|   IBIS model for TI AM261
[IBIS Ver]   5.1
[Disclaimer]   Please be aware that in the absence of a written agreement
|   Texas Instruments(TI) assumes no liability for:
|   (1) The accuracy of the IBIS models provided to your company,
|   however, the IBIS model is compliant to industry standard
|   IQ Level 2a.  Refer to IBIS Quality Section below for
|   for full details.
|   (2) The proper functioning of these Models in your design
|   or for any resulting applications
|   (3) Infringement of patents, copyrights or intellectual
|   property rights resulting from your use of these
|   models.
|   TI provides IBIS Models as a service to our customers and
|   therefore reserves the right to limit distribution of the
|   Models.  The information is subject to change without notice.
[File Name]  zfg.ibs
[File Rev]   0.1
|   -Initial version
|   -Updated Package model
[Date]   10 October 2024
[Source]   Texas Instruments Incorporated
[Copyright]   Property of Texas Instruments Incorporated.
|   Unauthorized reproduction and/or distribution is strictly.
|   prohibited.
|   This product is protected under copyright law and trade
|   secret law as an unpublished work.
|   Created 2012,(C) Copyright 1999-2012,
|   Texas Instruments Incorporated., All Rights Reserved.
|   These commodities are under the U.S. Government
|   distribution license control. As such,they are not to be
|   re-exported without the prior approval of the U.S.
|   Department of Commerce.
[Notes]
   ADC pins are marked as NC
   USB pins are marked as NC
   Clock pins are marked as NC
   nReset pin marked as NC
|   Revision History
|   GERNERAL COMMENT: All IBIS Quality Notes below reflect latest release
|   and version of IBIS File
|   File passes ibischk6.0 with 0 errors and 35 warnings
|   Component AM261
[Component] AM261
[Manufacturer] TEXAS INSTRUMENTS
[Package Model] AM261_ZFG
[Package]
|   typ   min   max
R_pkg   0.18633   0.087237   0.33822
L_pkg   3.165e-9   1.403e-9   5.371e-9
C_pkg   4.685e-13   3.303e-13   9.903e-13
[Pin]   Signal_name   model_name
F7   VDD   POWER
F9   VDD   POWER
F12   VDD   POWER
F14   VDD   POWER
G6   VDD   POWER
G15   VDD   POWER
J6   VDD   POWER
J15   VDD   POWER
M6   VDD   POWER
M15   VDD   POWER
P6   VDD   POWER
P15   VDD   POWER
R7   VDD   POWER
U10   VDDA18_LDO   POWER
U11   VDDA18_LDO   POWER
U8   VDDA18_OSC_PLL   POWER
T5   VDDA18_USB   POWER
T9   VDDA33   POWER
T12   VDDA33   POWER
P5   VDDA33_USB   POWER
D13   VDDAR2   POWER
H4   VDDAR3   POWER
E9   VDDS18   POWER
E14   VDDS18   POWER
F4   VDDS18   POWER
G16   VDDS18   POWER
L17   VDDS18   POWER
N4   VDDS18   POWER
T16   VDDS18   POWER
U6   VDDS18_LDO   POWER
E7   VDDSHV_A   POWER
E12   VDDSHV_A   POWER
E16   VDDSHV_A   POWER
G5   VDDSHV_A   POWER
J16   VDDSHV_A   POWER
M16   VDDSHV_A   POWER
M5   VDDSHV_B   POWER
T14   VDDSHV_C   POWER
J5   VDDSHV_D   POWER
P16   VDDSHV_E   POWER
T7   VDDSHV_F   POWER
V7   VDD_TEMP   NC
K17   VNWA   POWER
P3   VPP   POWER
W13   ADC0_AIN0   NC
U13   ADC0_AIN1   NC
W14   ADC0_AIN2   NC
V14   ADC0_AIN3   NC
Y14   ADC0_AIN4   NC
W15   ADC0_AIN5   NC
Y15   ADC0_AIN6   NC
W12   ADC1_AIN0   NC
V12   ADC1_AIN1   NC
Y11   ADC1_AIN2   NC
W11   ADC1_AIN3   NC
Y10   ADC1_AIN4   NC
W10   ADC1_AIN5   NC
W9   ADC1_AIN6   NC
W8   ADC2_AIN0   NC
Y7   ADC2_AIN1   NC
Y6   ADC2_AIN2   NC
W7   ADC2_AIN3   NC
W6   ADC2_AIN4   NC
V9   ADC2_AIN5   NC
Y5   ADC2_AIN6   NC
V16   ADC_CAL0   NC
Y12   ADC_VREFHI_G0   NC
Y8   ADC_VREFHI_G1   NC
Y13   ADC_VREFLO_G0   NC
Y9   ADC_VREFLO_G1   NC
W5   ATESTV1   NC
W4   DAC_OUT   NC
U15   DAC_VREF0   NC
U4   GPIO0   bc1833dv40dcpbfbp18ll_rxll_ssdlv
T2   GPIO1   bc1833dv40dcpbfbp18ll_rxll_ssdlv
M3   GPIO2   bc1833dv40dcpbfbp18ll_rxll_ssdlv
R2   GPIO3   bc1833dv40dcpbfbp18ll_ssdlv
R1   GPIO4   bc1833dv40dcpbfbp18ll_ssdlv
T1   GPIO5   bc1833dv40dcpbfbp18ll_rxll_ssdlv
U1   GPIO6   bc1833dv40dcpbfbp18ll_rxll_ssdlv
P1   GPIO7   bc1833dv40dcpbfbp18ll_rxll_ssdlv
P2   GPIO8   bc1833dv40dcpbfbp18ll_rxll_ssdlv
N2   GPIO9   bc1833dv40dcpbfbp18ll_rxll_ssdlv
N1   GPIO10   bc1833dv40dcpbfbp18ll_rxll_ssdlv
B13   GPIO11   bc1833dv40dcpbfbp18ll_rxll_ssdlh
A13   GPIO12   bc1833dv40dcpbfbp18ll_ssdlh
B12   GPIO13   bc1833dv40dcpbfbp18ll_ssdlh
C12   GPIO14   bc1833dv40dcpbfbp18ll_rxll_ssdlh
D11   GPIO15   bc1833dv40dcpbfbp18ll_rxll_ssdlh
A12   GPIO16   bc1833dv40dcpbfbp18ll_rxll_ssdlh
D10   GPIO17   bc1833dv40dcpbfbp18ll_rxll_ssdlh
C9   GPIO18   bc1833dv40dcpbfbp18ll_rxll_ssdlh
A11   GPIO19   bc1833dv40dcpbfbp18ll_rxll_ssdlh
B11   GPIO20   bc1833dv40dcpbfbp18ll_rxll_ssdlh
B10   GPIO21   bc1833dv40dcpbfbp18ll_rxll_ssdlh
A10   GPIO22   bc1833dv40dcpbfbp18ll_rxll_ssdlh
B9   GPIO23   bc1833dv40dcpbfbp18ll_rxll_ssdlh
A9   GPIO24   bc1833dv40dcpbfbp18ll_rxll_ssdlh
C7   GPIO25   bc1833dv40dcpbfbp18ll_rxll_ssdlh
D8   GPIO26   bc1833dv40dcpbfbp18ll_rxll_ssdlh
A8   GPIO27   bc1833dv40dcpbfbp18ll_rxll_ssdlh
B8   GPIO28   bc1833dv40dcpbfbp18ll_rxll_ssdlh
W20   GPIO29   bc1833dv40dcpbfbp18ll_rxll_ssdlv_135u
V19   GPIO30   bc1833dv40dcpbfbp18ll_rxll_ssdlv_135u
Y18   GPIO31   bc1833dv40dcpbfbp18ll_rxll_ssdlh
W18   GPIO32   bc1833dv40dcpbfbp18ll_rxll_ssdlh
Y19   GPIO33   bc1833dv40dcpbfbp18ll_rxll_ssdlh
W19   GPIO34   bc1833dv40dcpbfbp18ll_rxll_ssdlv_135u
U20   GPIO35   bc1833dv40dcpbfbp18ll_rxll_ssdlv_135u
T20   GPIO36   bc1833dv40dcpbfbp18ll_rxll_ssdlv_135u
V18   GPIO37   bc1833dv40dcpbfbp18ll_rxll_ssdlv_135u
V20   GPIO38   bc1833dv40dcpbfbp18ll_rxll_ssdlv_135u
U19   GPIO39   bc1833dv40dcpbfbp18ll_rxll_ssdlv_135u
T19   GPIO40   bc1833dv40dcpbfbp18ll_rxll_ssdlv_135u
R17   GPIO41   bc1833dv40dcpbfbp18ll_rxll_ssdlv_135u
T18   GPIO42   bc1833dv40dcpbfbp18ll_rxll_ssdlv_135u
B3   GPIO43   bc1833dv40dcpbfbp18ll_rxll_ssdlh_135u
C3   GPIO44   bc1833dv40dcpbfbp18ll_rxll_ssdlh_135u
A2   GPIO45   bc1833dv40dcpbfbp18ll_rxll_ssdlh_135u
A3   GPIO46   bc1833dv40dcpbfbp18ll_rxll_ssdlh_135u
B1   GPIO47   bc1833dv40dcpbfbp18ll_rxll_ssdlh_135u
B2   GPIO48   bc1833dv40dcpbfbp18ll_rxll_ssdlh_135u
C1   GPIO49   bc1833dv40dcpbfbp18ll_rxll_ssdlh_135u
C2   GPIO50   bc1833dv40dcpbfbp18ll_rxll_ssdlv
D2   GPIO51   bc1833dv40dcpbfbp18ll_rxll_ssdlv
D1   GPIO52   bc1833dv40dcpbfbp18ll_rxll_ssdlv
E2   GPIO53   bc1833dv40dcpbfbp18ll_rxll_ssdlv
E1   GPIO54   bc1833dv40dcpbfbp18ll_rxll_ssdlv
F2   GPIO55   bc1833dv40dcpbfbp18ll_rxll_ssdlv
F1   GPIO56   bc1833dv40dcpbfbp18ll_rxll_ssdlv
G2   GPIO57   bc1833dv40dcpbfbp18ll_rxll_ssdlv
G1   GPIO58   bc1833dv40dcpbfbp18ll_rxll_ssdlv
H2   GPIO59   bc1833dv40dcpbfbp18ll_rxll_ssdlv
H1   GPIO60   bc1833dv40dcpbfbp18ll_rxll_ssdlv
K4   GPIO61   bc1833dv40dcpbfbp18ll_rxll_ssdlv
L2   GPIO62   bc1833dv40dcpbfbp18ll_rxll_ssdlv
J2   GPIO63   bc1833dv40dcpbfbp18ll_rxll_ssdlv
J1   GPIO64   bc1833dv40dcpbfbp18ll_rxll_ssdlv
J3   GPIO65   bc1833dv40dcpbfbp18ll_rxll_ssdlv
K2   GPIO66   bc1833dv40dcpbfbp18ll_rxll_ssdlv
K1   GPIO67   bc1833dv40dcpbfbp18ll_rxll_ssdlv
L4   GPIO68   bc1833dv40dcpbfbp18ll_rxll_ssdlv
L1   GPIO69   bc1833dv40dcpbfbp18ll_rxll_ssdlv
M2   GPIO70   bc1833dv40dcpbfbp18ll_rxll_ssdlv
W16   GPIO71   bc1833dv40dcpbfbp18ll_rxll_ssdlh
Y16   GPIO72   bc1833dv40dcpbfbp18ll_rxll_ssdlh
W17   GPIO73   bc1833dv40dcpbfbp18ll_rxll_ssdlh
Y17   GPIO74   bc1833dv40dcpbfbp18ll_rxll_ssdlh
T3   GPIO75   bc1833dv40dcpbfbp18ll_rxll_ssdlv
R4   GPIO76   bc1833dv40dcpbfbp18ll_rxll_ssdlv
B7   GPIO77   bc1833dv40dcpbfbp18ll_rxll_ssdlh_135u
A6   GPIO78   bc1833dv40dcpbfbp18ll_rxll_ssdlh_135u
B6   GPIO79   bc1833dv40dcpbfbp18ll_rxll_ssdlh_135u
A5   GPIO80   bc1833dv40dcpbfbp18ll_rxll_ssdlh_135u
B5   GPIO81   bc1833dv40dcpbfbp18ll_rxll_ssdlh_135u
A4   GPIO82   bc1833dv40dcpbfbp18ll_rxll_ssdlh_135u
B4   GPIO83   bc1833dv40dcpbfbp18ll_rxll_ssdlh_135u
A7   GPIO84   bc1833dv40dcpbfbp18ll_rxll_ssdlh_135u
R19   GPIO85   bc1833dv40dcpbfbp18ll_rxll_ssdlv_135u
R20   GPIO86   bc1833dv40dcpbfbp18ll_rxll_ssdlv_135u
K19   GPIO87   bc1833dv40dcpbfbp18ll_rxll_ssdlv_135u
J19   GPIO88   bc1833dv40dcpbfbp18ll_rxll_ssdlv_135u
J20   GPIO89   bc1833dv40dcpbfbp18ll_rxll_ssdlv_135u
J18   GPIO90   bc1833dv40dcpbfbp18ll_rxll_ssdlv_135u
N20   GPIO91   bc1833dv40dcpbfbp18ll_rxll_ssdlv_135u
L20   GPIO92   bc1833dv40dcpbfbp18ll_rxll_ssdlv_135u
N17   GPIO93   bc1833dv40dcpbfbp18ll_rxll_ssdlv_135u
N19   GPIO94   bc1833dv40dcpbfbp18ll_rxll_ssdlv_135u
M18   GPIO95   bc1833dv40dcpbfbp18ll_rxll_ssdlv_135u
M20   GPIO96   bc1833dv40dcpbfbp18ll_rxll_ssdlv_135u
M19   GPIO97   bc1833dv40dcpbfbp18ll_rxll_ssdlv_135u
P18   GPIO98   bc1833dv40dcpbfbp18ll_rxll_ssdlv_135u
P20   GPIO99   bc1833dv40dcpbfbp18ll_rxll_ssdlv_135u
P19   GPIO100   bc1833dv40dcpbfbp18ll_rxll_ssdlv_135u
K20   GPIO101   bc1833dv40dcpbfbp18ll_rxll_ssdlv_135u
L19   GPIO102   bc1833dv40dcpbfbp18ll_rxll_ssdlv_135u
F20   GPIO103   bc1833dv40dcpbfbp18ll_rxll_ssdlv_135u
E20   GPIO104   bc1833dv40dcpbfbp18ll_rxll_ssdlv_135u
E19   GPIO105   bc1833dv40dcpbfbp18ll_rxll_ssdlv_135u
G18   GPIO106   bc1833dv40dcpbfbp18ll_rxll_ssdlv_135u
F19   GPIO107   bc1833dv40dcpbfbp18ll_rxll_ssdlv_135u
G19   GPIO108   bc1833dv40dcpbfbp18ll_rxll_ssdlv_135u
H20   GPIO109   bc1833dv40dcpbfbp18ll_rxll_ssdlv_135u
H19   GPIO110   bc1833dv40dcpbfbp18ll_rxll_ssdlv_135u
H17   GPIO111   bc1833dv40dcpbfbp18ll_rxll_ssdlv_135u
G20   GPIO112   bc1833dv40dcpbfbp18ll_rxll_ssdlv_135u
B20   GPIO113   bc1833dv40dcpbfbp18ll_rxll_ssdlv_135u
E18   GPIO114   bc1833dv40dcpbfbp18ll_rxll_ssdlv_135u
F17   GPIO115   bc1833dv40dcpbfbp18ll_rxll_ssdlv_135u
D20   GPIO116   bc1833dv40dcpbfbp18ll_rxll_ssdlv_135u
C20   GPIO117   bc1833dv40dcpbfbp18ll_rxll_ssdlv_135u
D19   GPIO118   bc1833dv40dcpbfbp18ll_rxll_ssdlv_135u
C18   GPIO119   bc1833dv40dcpbfbp18ll_rxll_ssdlh
C19   GPIO120   bc1833dv40dcpbfbp18ll_rxll_ssdlv_135u
U2   GPIO121   bc1833dv40dcpbfbp18ll_rxll_ssdlh
B19   GPIO122   bc1833dv40dcpbfbp18ll_rxll_ssdlh
C16   GPIO123   bc1833dv40dcpbfbp18ll_rxll_ssdlh
A19   GPIO124   bc1833dv40dcpbfbp18ll_rxll_ssdlh
B17   GPIO125   bc1833dv40dcpbfbp18ll_rxll_ssdlh
A18   GPIO126   bc1833dv40dcpbfbp18ll_rxll_ssdlh
A17   GPIO127   bc1833dv40dcpbfbp18ll_rxll_ssdlh
B18   GPIO128   bc1833dv40dcpbfbp18ll_rxll_ssdlh
D17   GPIO129   bc1833dv40dcpbfbp18ll_rxll_ssdlh
A16   GPIO130   bc1833dv40dcpbfbp18ll_rxll_ssdlh
B16   GPIO131   bc1833dv40dcpbfbp18ll_rxll_ssdlh
C14   GPIO132   bc1833dv40dcpbfbp18ll_rxll_ssdlh
D15   GPIO133   bc1833dv40dcpbfbp18ll_rxll_ssdlh
B15   GPIO134   bi2c1833dvfzp18_ssdlh
A15   GPIO135   bi2c1833dvfzp18_ssdlh
B14   GPIO136   bc1833dv40dcpbfbp18ll_rxll_ssdlv
A14   GPIO137   bc1833dv40dcpbfbp18ll_rxll_ssdlv
M1   GPIO138   bc1833dv40dcpbfbp18ll_rxll_ssdlv
V1   GPIO139   NC
W1   GPIO140   NC
V3   PORZ   ihhv1833dvhyp18ll_ssdhv
E3   SAFETY_ERRORN   bc1833dv40dcpbfbp18ll_ssdlh_135u
D4   TCK   iq1833dvtckpbfbp18ll_ssdhh_135u
C5   TDI   bc1833dv40dcpbfbp18ll_ssdlh_135u
E5   TDO   bc1833dv40dcpbfbp18ll_ssdlh_135u
W3   TEMPCAL   NC
D6   TMS   bc1833dv40dcpbfbp18ll_ssdlh_135u
Y4   VSYS_MON   NC
G3   WARMRSTN   bc1833dv40dcpbfbp18ll_od_fs_cmphdl_ssdlv
Y3   XTAL_XI   NC
Y2   XTAL_XO   NC
A1   VSS   GND
A20   VSS   GND
F6   VSS   GND
F15   VSS   GND
G7   VSS   GND
G8   VSS   GND
G9   VSS   GND
G10   VSS   GND
G11   VSS   GND
G12   VSS   GND
G13   VSS   GND
G14   VSS   GND
H7   VSS   GND
H8   VSS   GND
H9   VSS   GND
H10   VSS   GND
H11   VSS   GND
H12   VSS   GND
H13   VSS   GND
H14   VSS   GND
J7   VSS   GND
J8   VSS   GND
J9   VSS   GND
J10   VSS   GND
J11   VSS   GND
J12   VSS   GND
J13   VSS   GND
J14   VSS   GND
K7   VSS   GND
K8   VSS   GND
K9   VSS   GND
K10   VSS   GND
K11   VSS   GND
K12   VSS   GND
K13   VSS   GND
K14   VSS   GND
L7   VSS   GND
L8   VSS   GND
L9   VSS   GND
L10   VSS   GND
L11   VSS   GND
L12   VSS   GND
L13   VSS   GND
L14   VSS   GND
M7   VSS   GND
M8   VSS   GND
M9   VSS   GND
M10   VSS   GND
M11   VSS   GND
M12   VSS   GND
M13   VSS   GND
M14   VSS   GND
N7   VSS   GND
N8   VSS   GND
N9   VSS   GND
N10   VSS   GND
N11   VSS   GND
N12   VSS   GND
N13   VSS   GND
N14   VSS   GND
P7   VSS   GND
P8   VSS   GND
P9   VSS   GND
P10   VSS   GND
P11   VSS   GND
P12   VSS   GND
P13   VSS   GND
P14   VSS   GND
R6   VSS   GND
R14   VSS   GND
R15   VSS   GND
V2   VSS   GND
V5   VSS   GND
W2   VSS   GND
Y1   VSS   GND
Y20   VSS   GND
R9   VSSA   GND
R12   VSSA   GND
|   BC1833DV40DCPBFBP18LL_SSDLH
[Model Selector] bc1833dv40dcpbfbp18ll_ssdlh
|SC1 IS A SLEW RATE CONTROL PIN
|5% SUPPLY VARIATION MODES WITH 1.8V NOM SUPPLY
BC40D_H_PUPDOFF_5P_SC1_1P8  Cell operated at 1.8(nom)
|BC40D_H_PUPDOFF_5P_SC1_1P8; BUFFER WITH WEAK PULUP/PULLDOWN OFF AT 5% SUPPLY
|VARIATION WITH SC1=1 MEANING SLOW MODE OF OPERATION
BC40D_H_PD_ON_5P_!SC1_1P8  Cell operated at 1.8(nom)
|BC40D_H_PD_ON_5P_!SC1_1P8; BUFFER WITH WEAK_PULLDOWN_ON AT 5% SUPPLY
|VARIATION WITH SC1=0 MEANING FAST MODE OF OPERATION
BC40D_H_PD_ON_5P_SC1_1P8  Cell operated at 1.8(nom)
|BC40D_H_PD_ON_5P_SC1_1P8; BUFFER WITH WEAK_PULLDOWN_ON AT 5% SUPPLY
|VARIATION WITH SC1=1 MEANING SLOW MODE OF OPERATION
BC40D_H_PU_ON_5P_!SC1_1P8  Cell operated at 1.8(nom)
|BC40D_H_PU_ON_5P_!SC1_1P8; BUFFER WITH WEAK_PULLUP_ON AT 5% SUPPLY
|VARIATION WITH SC1=0 MEANING FAST MODE OF OPERATION
BC40D_H_PUPDOFF_5P_!SC1_1P8  Cell operated at 1.8(nom)
|BC40D_H_PUPDOFF_5P_!SC1_1P8; BUFFER WITH WEAK PULUP/PULLDOWN OFF AT 5% SUPPLY
|VARIATION WITH SC1=0 MEANING FAST MODE OF OPERATION
BC40D_H_PU_ON_5P_SC1_1P8  Cell operated at 1.8(nom)
|BC40D_H_PU_ON_5P_SC1_1P8; BUFFER WITH WEAK_PULLUP_ON AT 5% SUPPLY
|VARIATION WITH SC1=1 MEANING SLOW MODE OF OPERATION
|5% SUPPLY VARIATION MODES WITH 3.3V NOM SUPPLY
BC40D_H_PUPDOFF_5P_SC1_3P3  Cell operated at 3.3(nom)
|BC40D_H_PUPDOFF_5P_SC1_3P3; BUFFER WITH WEAK PULUP/PULLDOWN OFF AT 5% SUPPLY
|VARIATION WITH SC1=1 MEANING SLOW MODE OF OPERATION
BC40D_H_PD_ON_5P_!SC1_3P3  Cell operated at 3.3(nom)
|BC40D_H_PD_ON_5P_!SC1_3P3; BUFFER WITH WEAK_PULLDOWN_ON AT 5% SUPPLY
|VARIATION WITH SC1=0 MEANING FAST MODE OF OPERATION
BC40D_H_PD_ON_5P_SC1_3P3  Cell operated at 3.3(nom)
|BC40D_H_PD_ON_5P_SC1_3P3; BUFFER WITH WEAK_PULLDOWN_ON AT 5% SUPPLY
|VARIATION WITH SC1=1 MEANING SLOW MODE OF OPERATION
BC40D_H_PU_ON_5P_!SC1_3P3  Cell operated at 3.3(nom)
|BC40D_H_PU_ON_5P_!SC1_3P3; BUFFER WITH WEAK_PULLUP_ON AT 5% SUPPLY
|VARIATION WITH SC1=0 MEANING FAST MODE OF OPERATION
BC40D_H_PUPDOFF_5P_!SC1_3P3  Cell operated at 3.3(nom)
|BC40D_H_PUPDOFF_5P_!SC1_3P3; BUFFER WITH WEAK PULUP/PULLDOWN OFF AT 5% SUPPLY
|VARIATION WITH SC1=0 MEANING FAST MODE OF OPERATION
BC40D_H_PU_ON_5P_SC1_3P3  Cell operated at 3.3(nom)
|BC40D_H_PU_ON_5P_SC1_3P3; BUFFER WITH WEAK_PULLUP_ON AT 5% SUPPLY
|VARIATION WITH SC1=1 MEANING SLOW MODE OF OPERATION
| 10% SUPPLY VARIATION MODES WITH 1.8V NOM SUPPLY
BC40D_H_PUPDOFF_10P_SC1_1P8  Cell operated at 1.8(nom)
|BC40D_H_PUPDOFF_10P_SC1_1P8; BUFFER WITH WEAK PULUP/PULLDOWN OFF AT 10% SUPPLY
|VARIATION WITH SC1=1 MEANING SLOW MODE OF OPERATION
BC40D_H_PD_ON_10P_!SC1_1P8  Cell operated at 1.8(nom)
|BC40D_H_PD_ON_10P_!SC1_1P8; BUFFER WITH WEAK_PULLDOWN_ON AT 10% SUPPLY
|VARIATION WITH SC1=0 MEANING FAST MODE OF OPERATION
BC40D_H_PD_ON_10P_SC1_1P8  Cell operated at 1.8(nom)
|BC40D_H_PD_ON_10P_SC1_1P8; BUFFER WITH WEAK_PULLDOWN_ON AT 10% SUPPLY
|VARIATION WITH SC1=1 MEANING SLOW MODE OF OPERATION
BC40D_H_PU_ON_10P_!SC1_1P8  Cell operated at 1.8(nom)
|BC40D_H_PU_ON_10P_!SC1_1P8; BUFFER WITH WEAK_PULLUP_ON AT 10% SUPPLY
|VARIATION WITH SC1=0 MEANING FAST MODE OF OPERATION
BC40D_H_PUPDOFF_10P_!SC1_1P8  Cell operated at 1.8(nom)
|BC40D_H_PUPDOFF_10P_!SC1_1P8; BUFFER WITH WEAK PULUP/PULLDOWN OFF AT 10% SUPPLY
|VARIATION WITH SC1=0 MEANING FAST MODE OF OPERATION
BC40D_H_PU_ON_10P_SC1_1P8  Cell operated at 1.8(nom)
|BC40D_H_PU_ON_10P_SC1_1P8; BUFFER WITH WEAK_PULLUP_ON AT 10% SUPPLY
|VARIATION WITH SC1=1 MEANING SLOW MODE OF OPERATION
| 10% SUPPLY VARIATION MODES WITH 3.3V NOM SUPPLY
BC40D_H_PUPDOFF_10P_SC1_3P3  Cell operated at 3.3(nom)
|BC40D_H_PUPDOFF_10P_SC1_3P3; BUFFER WITH WEAK PULUP/PULLDOWN OFF AT 10% SUPPLY
|VARIATION WITH SC1=1 MEANING SLOW MODE OF OPERATION
BC40D_H_PD_ON_10P_!SC1_3P3  Cell operated at 3.3(nom)
|BC40D_H_PD_ON_10P_!SC1_3P3; BUFFER WITH WEAK_PULLDOWN_ON 10% SUPPLY
|VARIATION WITH SC1=0 MEANING FAST MODE OF OPERATION
BC40D_H_PD_ON_10P_SC1_3P3  Cell operated at 3.3(nom)
|BC40D_H_PD_ON_10P_SC1_3P3; BUFFER WITH WEAK_PULLDOWN_ON AT 10% SUPPLY
|VARIATION WITH SC1=1 MEANING SLOW MODE OF OPERATION
BC40D_H_PU_ON_10P_!SC1_3P3  Cell operated at 3.3(nom)
|BC40D_H_PU_ON_10P_!SC1_3P3; BUFFER WITH WEAK_PULLUP_ON AT 10% SUPPLY
|VARIATION WITH SC1=0 MEANING FAST MODE OF OPERATION
BC40D_H_PUPDOFF_10P_!SC1_3P3  Cell operated at 3.3(nom)
|BC40D_H_PUPDOFF_10P_!SC1_3P3; BUFFER WITH WEAK PULUP/PULLDOWN OFF AT 10% SUPPLY
|VARIATION WITH SC1=0 MEANING FAST MODE OF OPERATION
BC40D_H_PU_ON_10P_SC1_3P3  Cell operated at 3.3(nom)
|BC40D_H_PU_ON_10P_SC1_3P3; BUFFER WITH WEAK_PULLUP_ON AT 10% SUPPLY
|VARIATION WITH SC1=1 MEANING SLOW MODE OF OPERATION
|   BC1833DV40DCPBFBP18LL_SSDLV
[Model Selector] bc1833dv40dcpbfbp18ll_ssdlv
|SC1 IS A SLEW RATE CONTROL PIN
|5% SUPPLY VARIATION MODES WITH 1.8V NOM SUPPLY
BC40D_V_PUPDOFF_5P_SC1_1P8  Cell operated at 1.8(nom)
|BC40D_V_PUPDOFF_5P_SC1_1P8; BUFFER WITH WEAK PULUP/PULLDOWN OFF AT 5% SUPPLY
|VARIATION WITH SC1=1 MEANING SLOW MODE OF OPERATION
BC40D_V_PD_ON_5P_!SC1_1P8  Cell operated at 1.8(nom)
|BC40D_V_PD_ON_5P_!SC1_1P8; BUFFER WITH WEAK_PULLDOWN_ON AT 5% SUPPLY
|VARIATION WITH SC1=0 MEANING FAST MODE OF OPERATION
BC40D_V_PD_ON_5P_SC1_1P8  Cell operated at 1.8(nom)
|BC40D_V_PD_ON_5P_SC1_1P8; BUFFER WITH WEAK_PULLDOWN_ON AT 5% SUPPLY
|VARIATION WITH SC1=1 MEANING SLOW MODE OF OPERATION
BC40D_V_PU_ON_5P_!SC1_1P8  Cell operated at 1.8(nom)
|BC40D_V_PU_ON_5P_!SC1_1P8; BUFFER WITH WEAK_PULLUP_ON AT 5% SUPPLY
|VARIATION WITH SC1=0 MEANING FAST MODE OF OPERATION
BC40D_V_PUPDOFF_5P_!SC1_1P8  Cell operated at 1.8(nom)
|BC40D_V_PUPDOFF_5P_!SC1_1P8; BUFFER WITH WEAK PULUP/PULLDOWN OFF AT 5% SUPPLY
|VARIATION WITH SC1=0 MEANING FAST MODE OF OPERATION
BC40D_V_PU_ON_5P_SC1_1P8  Cell operated at 1.8(nom)
|BC40D_V_PU_ON_5P_SC1_1P8; BUFFER WITH WEAK_PULLUP_ON AT 5% SUPPLY
|VARIATION WITH SC1=1 MEANING SLOW MODE OF OPERATION
|5% SUPPLY VARIATION MODES WITH 3.3V NOM SUPPLY
BC40D_V_PUPDOFF_5P_SC1_3P3  Cell operated at 3.3(nom)
|BC40D_V_PUPDOFF_5P_SC1_3P3; BUFFER WITH WEAK PULUP/PULLDOWN OFF AT 5% SUPPLY
|VARIATION WITH SC1=1 MEANING SLOW MODE OF OPERATION
BC40D_V_PD_ON_5P_!SC1_3P3  Cell operated at 3.3(nom)
|BC40D_V_PD_ON_5P_!SC1_3P3; BUFFER WITH WEAK_PULLDOWN_ON AT 5% SUPPLY
|VARIATION WITH SC1=0 MEANING FAST MODE OF OPERATION
BC40D_V_PD_ON_5P_SC1_3P3  Cell operated at 3.3(nom)
|BC40D_V_PD_ON_5P_SC1_3P3; BUFFER WITH WEAK_PULLDOWN_ON AT 5% SUPPLY
|VARIATION WITH SC1=1 MEANING SLOW MODE OF OPERATION
BC40D_V_PU_ON_5P_!SC1_3P3  Cell operated at 3.3(nom)
|BC40D_V_PU_ON_5P_!SC1_3P3; BUFFER WITH WEAK_PULLUP_ON AT 5% SUPPLY
|VARIATION WITH SC1=0 MEANING FAST MODE OF OPERATION
BC40D_V_PUPDOFF_5P_!SC1_3P3  Cell operated at 3.3(nom)
|BC40D_V_PUPDOFF_5P_!SC1_3P3; BUFFER WITH WEAK PULUP/PULLDOWN OFF AT 5% SUPPLY
|VARIATION WITH SC1=0 MEANING FAST MODE OF OPERATION
BC40D_V_PU_ON_5P_SC1_3P3  Cell operated at 3.3(nom)
|BC40D_V_PU_ON_5P_SC1_3P3; BUFFER WITH WEAK_PULLUP_ON AT 5% SUPPLY
|VARIATION WITH SC1=1 MEANING SLOW MODE OF OPERATION
| 10% SUPPLY VARIATION MODES WITH 1.8V NOM SUPPLY
BC40D_V_PUPDOFF_10P_SC1_1P8  Cell operated at 1.8(nom)
|BC40D_V_PUPDOFF_10P_SC1_1P8; BUFFER WITH WEAK PULUP/PULLDOWN OFF AT 10% SUPPLY
|VARIATION WITH SC1=1 MEANING SLOW MODE OF OPERATION
BC40D_V_PD_ON_10P_!SC1_1P8  Cell operated at 1.8(nom)
|BC40D_V_PD_ON_10P_!SC1_1P8; BUFFER WITH WEAK_PULLDOWN_ON AT 10% SUPPLY
|VARIATION WITH SC1=0 MEANING FAST MODE OF OPERATION
BC40D_V_PD_ON_10P_SC1_1P8  Cell operated at 1.8(nom)
|BC40D_V_PD_ON_10P_SC1_1P8; BUFFER WITH WEAK_PULLDOWN_ON AT 10% SUPPLY
|VARIATION WITH SC1=1 MEANING SLOW MODE OF OPERATION
BC40D_V_PU_ON_10P_!SC1_1P8  Cell operated at 1.8(nom)
|BC40D_V_PU_ON_10P_!SC1_1P8; BUFFER WITH WEAK_PULLUP_ON AT 10% SUPPLY
|VARIATION WITH SC1=0 MEANING FAST MODE OF OPERATION
BC40D_V_PUPDOFF_10P_!SC1_1P8  Cell operated at 1.8(nom)
|BC40D_V_PUPDOFF_10P_!SC1_1P8; BUFFER WITH WEAK PULUP/PULLDOWN OFF AT 10% SUPPLY
|VARIATION WITH SC1=0 MEANING FAST MODE OF OPERATION
BC40D_V_PU_ON_10P_SC1_1P8  Cell operated at 1.8(nom)
|BC40D_V_PU_ON_10P_SC1_1P8; BUFFER WITH WEAK_PULLUP_ON AT 10% SUPPLY
|VARIATION WITH SC1=1 MEANING SLOW MODE OF OPERATION
| 10% SUPPLY VARIATION MODES WITH 3.3V NOM SUPPLY
BC40D_V_PUPDOFF_10P_SC1_3P3  Cell operated at 3.3(nom)
|BC40D_V_PUPDOFF_10P_SC1_3P3; BUFFER WITH WEAK PULUP/PULLDOWN OFF AT 10% SUPPLY
|VARIATION WITH SC1=1 MEANING SLOW MODE OF OPERATION
BC40D_V_PD_ON_10P_!SC1_3P3  Cell operated at 3.3(nom)
|BC40D_V_PD_ON_10P_!SC1_3P3; BUFFER WITH WEAK_PULLDOWN_ON 10% SUPPLY
|VARIATION WITH SC1=0 MEANING FAST MODE OF OPERATION
BC40D_V_PD_ON_10P_SC1_3P3  Cell operated at 3.3(nom)
|BC40D_V_PD_ON_10P_SC1_3P3; BUFFER WITH WEAK_PULLDOWN_ON AT 10% SUPPLY
|VARIATION WITH SC1=1 MEANING SLOW MODE OF OPERATION
BC40D_V_PU_ON_10P_!SC1_3P3  Cell operated at 3.3(nom)
|BC40D_V_PU_ON_10P_!SC1_3P3; BUFFER WITH WEAK_PULLUP_ON AT 10% SUPPLY
|VARIATION WITH SC1=0 MEANING FAST MODE OF OPERATION
BC40D_V_PUPDOFF_10P_!SC1_3P3  Cell operated at 3.3(nom)
|BC40D_V_PUPDOFF_10P_!SC1_3P3; BUFFER WITH WEAK PULUP/PULLDOWN OFF AT 10% SUPPLY
|VARIATION WITH SC1=0 MEANING FAST MODE OF OPERATION
BC40D_V_PU_ON_10P_SC1_3P3  Cell operated at 3.3(nom)
|BC40D_V_PU_ON_10P_SC1_3P3; BUFFER WITH WEAK_PULLUP_ON AT 10% SUPPLY
|VARIATION WITH SC1=1 MEANING SLOW MODE OF OPERATION
|   BI2C1833DVFZP18_SSDLH
[Model Selector] bi2c1833dvfzp18_ssdlh
BI2C1833_NORAML_5P_1P8  Cell operated at 1.8(nom)
|BI2C1833_NORAML_5P_1P8; I2C MODE AT 1.8V WITH 5% SUPPLY VARIATION
BI2C1833_NORAML_5P_3P3  Cell operated at 3.3(nom)
|BI2C1833_NORAML_5P_3P3; I2C MODE AT 3.3V WITH 5% SUPPLY VARIATION
BI2C1833_NORAML_10P_1P8  Cell operated at 1.8(nom)
|BI2C1833_NORAML_10P_1P8; I2C MODE AT 1.8V WITH 10% SUPPLY VARIATION
BI2C1833_NORAML_10P_3P3  Cell operated at 3.3(nom)
|BI2C1833_NORAML_10P_3P3; I2C MODE AT 3.3V WITH 10% SUPPLY VARIATION
|   IHHV1833DVHYP18LL_SSDHV
[Model Selector] ihhv1833dvhyp18ll_ssdhv
IHHV_NORAML_5P_1P8  Cell operated at 1.8(nom)
|IHHV_NORAML_5P_1P8; NORMAL MODE AT 1.8V WITH 5% SUPPLY VARIATION
IHHV_NORAML_5P_3P3  Cell operated at 3.3(nom)
|IHHV_NORAML_5P_3P3; NORMAL MODE AT 3.3V WITH 5% SUPPLY VARIATION
IHHV_NORAML_10P_1P8  Cell operated at 1.8(nom)
|IHHV_NORAML_10P_1P8; NORMAL MODE AT 1.8V WITH 10% SUPPLY VARIATION
IHHV_NORAML_10P_3P3  Cell operated at 3.3(nom)
|IHHV_NORAML_10P_3P3; NORMAL MODE AT 3.3V WITH 10% SUPPLY VARIATION
|   BC1833DV40DCPBFBP18LL_OD_FS_CSTMPHOLDL_SSDLV
[Model Selector] bc1833dv40dcpbfbp18ll_od_fs_cmphdl_ssdlv
|SC1 IS A SLEW RATE CONTROL PIN
|5% SUPPLY VARIATION MODES WITH 1.8V NOM SUPPLY
BC40D_V_PUPDOFF_5P_SC1_1P8  Cell operated at 1.8(nom)
|BC40D_V_PUPDOFF_5P_SC1_1P8; BUFFER WITH WEAK PULUP/PULLDOWN OFF AT 5% SUPPLY
|VARIATION WITH SC1=1 MEANING SLOW MODE OF OPERATION
BC40D_V_PD_ON_5P_!SC1_1P8  Cell operated at 1.8(nom)
|BC40D_V_PD_ON_5P_!SC1_1P8; BUFFER WITH WEAK_PULLDOWN_ON AT 5% SUPPLY
|VARIATION WITH SC1=0 MEANING FAST MODE OF OPERATION
BC40D_V_PD_ON_5P_SC1_1P8  Cell operated at 1.8(nom)
|BC40D_V_PD_ON_5P_SC1_1P8; BUFFER WITH WEAK_PULLDOWN_ON AT 5% SUPPLY
|VARIATION WITH SC1=1 MEANING SLOW MODE OF OPERATION
BC40D_V_PU_ON_5P_!SC1_1P8  Cell operated at 1.8(nom)
|BC40D_V_PU_ON_5P_!SC1_1P8; BUFFER WITH WEAK_PULLUP_ON AT 5% SUPPLY
|VARIATION WITH SC1=0 MEANING FAST MODE OF OPERATION
BC40D_V_PUPDOFF_5P_!SC1_1P8  Cell operated at 1.8(nom)
|BC40D_V_PUPDOFF_5P_!SC1_1P8; BUFFER WITH WEAK PULUP/PULLDOWN OFF AT 5% SUPPLY
|VARIATION WITH SC1=0 MEANING FAST MODE OF OPERATION
BC40D_V_PU_ON_5P_SC1_1P8  Cell operated at 1.8(nom)
|BC40D_V_PU_ON_5P_SC1_1P8; BUFFER WITH WEAK_PULLUP_ON AT 5% SUPPLY
|VARIATION WITH SC1=1 MEANING SLOW MODE OF OPERATION
|5% SUPPLY VARIATION MODES WITH 3.3V NOM SUPPLY
BC40D_V_PUPDOFF_5P_SC1_3P3  Cell operated at 3.3(nom)
|BC40D_V_PUPDOFF_5P_SC1_3P3; BUFFER WITH WEAK PULUP/PULLDOWN OFF AT 5% SUPPLY
|VARIATION WITH SC1=1 MEANING SLOW MODE OF OPERATION
BC40D_V_PD_ON_5P_!SC1_3P3  Cell operated at 3.3(nom)
|BC40D_V_PD_ON_5P_!SC1_3P3; BUFFER WITH WEAK_PULLDOWN_ON AT 5% SUPPLY
|VARIATION WITH SC1=0 MEANING FAST MODE OF OPERATION
BC40D_V_PD_ON_5P_SC1_3P3  Cell operated at 3.3(nom)
|BC40D_V_PD_ON_5P_SC1_3P3; BUFFER WITH WEAK_PULLDOWN_ON AT 5% SUPPLY
|VARIATION WITH SC1=1 MEANING SLOW MODE OF OPERATION
BC40D_V_PU_ON_5P_!SC1_3P3  Cell operated at 3.3(nom)
|BC40D_V_PU_ON_5P_!SC1_3P3; BUFFER WITH WEAK_PULLUP_ON AT 5% SUPPLY
|VARIATION WITH SC1=0 MEANING FAST MODE OF OPERATION
BC40D_V_PUPDOFF_5P_!SC1_3P3  Cell operated at 3.3(nom)
|BC40D_V_PUPDOFF_5P_!SC1_3P3; BUFFER WITH WEAK PULUP/PULLDOWN OFF AT 5% SUPPLY
|VARIATION WITH SC1=0 MEANING FAST MODE OF OPERATION
BC40D_V_PU_ON_5P_SC1_3P3  Cell operated at 3.3(nom)
|BC40D_V_PU_ON_5P_SC1_3P3; BUFFER WITH WEAK_PULLUP_ON AT 5% SUPPLY
|VARIATION WITH SC1=1 MEANING SLOW MODE OF OPERATION
| 10% SUPPLY VARIATION MODES WITH 1.8V NOM SUPPLY
BC40D_V_PUPDOFF_10P_SC1_1P8  Cell operated at 1.8(nom)
|BC40D_V_PUPDOFF_10P_SC1_1P8; BUFFER WITH WEAK PULUP/PULLDOWN OFF AT 10% SUPPLY
|VARIATION WITH SC1=1 MEANING SLOW MODE OF OPERATION
BC40D_V_PD_ON_10P_!SC1_1P8  Cell operated at 1.8(nom)
|BC40D_V_PD_ON_10P_!SC1_1P8; BUFFER WITH WEAK_PULLDOWN_ON AT 10% SUPPLY
|VARIATION WITH SC1=0 MEANING FAST MODE OF OPERATION
BC40D_V_PD_ON_10P_SC1_1P8  Cell operated at 1.8(nom)
|BC40D_V_PD_ON_10P_SC1_1P8; BUFFER WITH WEAK_PULLDOWN_ON AT 10% SUPPLY
|VARIATION WITH SC1=1 MEANING SLOW MODE OF OPERATION
BC40D_V_PU_ON_10P_!SC1_1P8  Cell operated at 1.8(nom)
|BC40D_V_PU_ON_10P_!SC1_1P8; BUFFER WITH WEAK_PULLUP_ON AT 10% SUPPLY
|VARIATION WITH SC1=0 MEANING FAST MODE OF OPERATION
BC40D_V_PUPDOFF_10P_!SC1_1P8  Cell operated at 1.8(nom)
|BC40D_V_PUPDOFF_10P_!SC1_1P8; BUFFER WITH WEAK PULUP/PULLDOWN OFF AT 10% SUPPLY
|VARIATION WITH SC1=0 MEANING FAST MODE OF OPERATION
BC40D_V_PU_ON_10P_SC1_1P8  Cell operated at 1.8(nom)
|BC40D_V_PU_ON_10P_SC1_1P8; BUFFER WITH WEAK_PULLUP_ON AT 10% SUPPLY
|VARIATION WITH SC1=1 MEANING SLOW MODE OF OPERATION
| 10% SUPPLY VARIATION MODES WITH 3.3V NOM SUPPLY
BC40D_V_PUPDOFF_10P_SC1_3P3  Cell operated at 3.3(nom)
|BC40D_V_PUPDOFF_10P_SC1_3P3; BUFFER WITH WEAK PULUP/PULLDOWN OFF AT 10% SUPPLY
|VARIATION WITH SC1=1 MEANING SLOW MODE OF OPERATION
BC40D_V_PD_ON_10P_!SC1_3P3  Cell operated at 3.3(nom)
|BC40D_V_PD_ON_10P_!SC1_3P3; BUFFER WITH WEAK_PULLDOWN_ON 10% SUPPLY
|VARIATION WITH SC1=0 MEANING FAST MODE OF OPERATION
BC40D_V_PD_ON_10P_SC1_3P3  Cell operated at 3.3(nom)
|BC40D_V_PD_ON_10P_SC1_3P3; BUFFER WITH WEAK_PULLDOWN_ON AT 10% SUPPLY
|VARIATION WITH SC1=1 MEANING SLOW MODE OF OPERATION
BC40D_V_PU_ON_10P_!SC1_3P3  Cell operated at 3.3(nom)
|BC40D_V_PU_ON_10P_!SC1_3P3; BUFFER WITH WEAK_PULLUP_ON AT 10% SUPPLY
|VARIATION WITH SC1=0 MEANING FAST MODE OF OPERATION
BC40D_V_PUPDOFF_10P_!SC1_3P3  Cell operated at 3.3(nom)
|BC40D_V_PUPDOFF_10P_!SC1_3P3; BUFFER WITH WEAK PULUP/PULLDOWN OFF AT 10% SUPPLY
|VARIATION WITH SC1=0 MEANING FAST MODE OF OPERATION
BC40D_V_PU_ON_10P_SC1_3P3  Cell operated at 3.3(nom)
|BC40D_V_PU_ON_10P_SC1_3P3; BUFFER WITH WEAK_PULLUP_ON AT 10% SUPPLY
|VARIATION WITH SC1=1 MEANING SLOW MODE OF OPERATION
|   IQ1833DVTCKPBFBP18LL_SSDHH_135U
[Model Selector] iq1833dvtckpbfbp18ll_ssdhh_135u
|5% SUPPLY VARIATION MODES WITH 1.8V NOM SUPPLY
IQ_SSDHH_PD_ON_5P_1P8  Cell operated at 1.8(nom)
|IQ_SSDHH_PD_ON_5P_1P8; BUFFER WITH WEAK_PULLDOWN_ON AT 5% SUPPLY VARIATION
IQ_SSDHH_PU_ON_5P_1P8  Cell operated at 1.8(nom)
|IQ_SSDHH_PU_ON_5P_1P8; BUFFER WITH WEAK_PULLUP_ON AT 5% SUPPLY VARIATION
IQ_SSDHH_PUPDOFF_5P_1P8  Cell operated at 1.8(nom)
|IQ_SSDHH_PUPDOFF_5P_1P8; BUFFER WITH WEAK PUPD OFF AT 5% SUPPLY VARIATION
|5% SUPPLY VARIATION MODES WITH 3.3V NOM SUPPLY
IQ_SSDHH_PD_ON_5P_3P3  Cell operated at 3.3(nom)
|IQ_SSDHH_PD_ON_5P_3P3; BUFFER WITH WEAK_PULLDOWN_ON AT 5% SUPPLY VARIATION
IQ_SSDHH_PU_ON_5P_3P3  Cell operated at 3.3(nom)
|IQ_SSDHH_PU_ON_5P_3P3; BUFFER WITH WEAK_PULLUP_ON AT 5% SUPPLY VARIATION
IQ_SSDHH_PUPDOFF_5P_3P3  Cell operated at 3.3(nom)
|IQ_SSDHH_PUPDOFF_5P_3P3; BUFFER WITH WEAK PUPD OFF AT 5% SUPPLY VARIATION
|10% SUPPLY VARIATION MODES WITH 1.8V NOM SUPPLY
IQ_SSDHH_PD_ON_10P_1P8  Cell operated at 1.8(nom)
|IQ_SSDHH_PD_ON_10P_1P8; BUFFER WITH WEAK_PULLDOWN_ON AT 10% SUPPLY VARIATION
IQ_SSDHH_PU_ON_10P_1P8  Cell operated at 1.8(nom)
|IQ_SSDHH_PU_ON_10P_1P8; BUFFER WITH WEAK_PULLUP_ON AT 10% SUPPLY VARIATION
IQ_SSDHH_PUPDOFF_10P_1P8  Cell operated at 1.8(nom)
|IQ_SSDHH_PUPDOFF_10P_1P8; BUFFER WITH WEAK PUPD OFF AT 10% SUPPLY VARIATION
|10% SUPPLY VARIATION MODES WITH 3.3V NOM SUPPLY
IQ_SSDHH_PD_ON_10P_3P3  Cell operated at 3.3(nom)
|IQ_SSDHH_PD_ON_10P_3P3; BUFFER WITH WEAK_PULLDOWN_ON  AT 10% SUPPLY VARIATION
IQ_SSDHH_PU_ON_10P_3P3  Cell operated at 3.3(nom)
|IQ_SSDHH_PU_ON_10P_3P3; BUFFER WITH WEAK_PULLUP_ON AT 10% SUPPLY VARIATION
IQ_SSDHH_PUPDOFF_10P_3P3  Cell operated at 3.3(nom)
|IQ_SSDHH_PUPDOFF_10P_3P3; BUFFER WITH WEAK PUPD OFF AT 10% SUPPLY VARIATION
|   BC1833DV40DCPBFBP18LL_RXLL_SSDLH
[Model Selector] bc1833dv40dcpbfbp18ll_rxll_ssdlh
|SC1 IS A SLEW RATE CONTROL PIN
|5% SUPPLY VARIATION MODES WITH 1.8V NOM SUPPLY
BC40D_H_PUPDOFF_5P_SC1_1P8  Cell operated at 1.8(nom)
|BC40D_H_PUPDOFF_5P_SC1_1P8; BUFFER WITH WEAK PULUP/PULLDOWN OFF AT 5% SUPPLY
|VARIATION WITH SC1=1 MEANING SLOW MODE OF OPERATION
BC40D_H_PD_ON_5P_!SC1_1P8  Cell operated at 1.8(nom)
|BC40D_H_PD_ON_5P_!SC1_1P8; BUFFER WITH WEAK_PULLDOWN_ON AT 5% SUPPLY
|VARIATION WITH SC1=0 MEANING FAST MODE OF OPERATION
BC40D_H_PD_ON_5P_SC1_1P8  Cell operated at 1.8(nom)
|BC40D_H_PD_ON_5P_SC1_1P8; BUFFER WITH WEAK_PULLDOWN_ON AT 5% SUPPLY
|VARIATION WITH SC1=1 MEANING SLOW MODE OF OPERATION
BC40D_H_PU_ON_5P_!SC1_1P8  Cell operated at 1.8(nom)
|BC40D_H_PU_ON_5P_!SC1_1P8; BUFFER WITH WEAK_PULLUP_ON AT 5% SUPPLY
|VARIATION WITH SC1=0 MEANING FAST MODE OF OPERATION
BC40D_H_PUPDOFF_5P_!SC1_1P8  Cell operated at 1.8(nom)
|BC40D_H_PUPDOFF_5P_!SC1_1P8; BUFFER WITH WEAK PULUP/PULLDOWN OFF AT 5% SUPPLY
|VARIATION WITH SC1=0 MEANING FAST MODE OF OPERATION
BC40D_H_PU_ON_5P_SC1_1P8  Cell operated at 1.8(nom)
|BC40D_H_PU_ON_5P_SC1_1P8; BUFFER WITH WEAK_PULLUP_ON AT 5% SUPPLY
|VARIATION WITH SC1=1 MEANING SLOW MODE OF OPERATION
|5% SUPPLY VARIATION MODES WITH 3.3V NOM SUPPLY
BC40D_H_PUPDOFF_5P_SC1_3P3  Cell operated at 3.3(nom)
|BC40D_H_PUPDOFF_5P_SC1_3P3; BUFFER WITH WEAK PULUP/PULLDOWN OFF AT 5% SUPPLY
|VARIATION WITH SC1=1 MEANING SLOW MODE OF OPERATION
BC40D_H_PD_ON_5P_!SC1_3P3  Cell operated at 3.3(nom)
|BC40D_H_PD_ON_5P_!SC1_3P3; BUFFER WITH WEAK_PULLDOWN_ON AT 5% SUPPLY
|VARIATION WITH SC1=0 MEANING FAST MODE OF OPERATION
BC40D_H_PD_ON_5P_SC1_3P3  Cell operated at 3.3(nom)
|BC40D_H_PD_ON_5P_SC1_3P3; BUFFER WITH WEAK_PULLDOWN_ON AT 5% SUPPLY
|VARIATION WITH SC1=1 MEANING SLOW MODE OF OPERATION
BC40D_H_PU_ON_5P_!SC1_3P3  Cell operated at 3.3(nom)
|BC40D_H_PU_ON_5P_!SC1_3P3; BUFFER WITH WEAK_PULLUP_ON AT 5% SUPPLY
|VARIATION WITH SC1=0 MEANING FAST MODE OF OPERATION
BC40D_H_PUPDOFF_5P_!SC1_3P3  Cell operated at 3.3(nom)
|BC40D_H_PUPDOFF_5P_!SC1_3P3; BUFFER WITH WEAK PULUP/PULLDOWN OFF AT 5% SUPPLY
|VARIATION WITH SC1=0 MEANING FAST MODE OF OPERATION
BC40D_H_PU_ON_5P_SC1_3P3  Cell operated at 3.3(nom)
|BC40D_H_PU_ON_5P_SC1_3P3; BUFFER WITH WEAK_PULLUP_ON AT 5% SUPPLY
|VARIATION WITH SC1=1 MEANING SLOW MODE OF OPERATION
| 10% SUPPLY VARIATION MODES WITH 1.8V NOM SUPPLY
BC40D_H_PUPDOFF_10P_SC1_1P8  Cell operated at 1.8(nom)
|BC40D_H_PUPDOFF_10P_SC1_1P8; BUFFER WITH WEAK PULUP/PULLDOWN OFF AT 10% SUPPLY
|VARIATION WITH SC1=1 MEANING SLOW MODE OF OPERATION
BC40D_H_PD_ON_10P_!SC1_1P8  Cell operated at 1.8(nom)
|BC40D_H_PD_ON_10P_!SC1_1P8; BUFFER WITH WEAK_PULLDOWN_ON AT 10% SUPPLY
|VARIATION WITH SC1=0 MEANING FAST MODE OF OPERATION
BC40D_H_PD_ON_10P_SC1_1P8  Cell operated at 1.8(nom)
|BC40D_H_PD_ON_10P_SC1_1P8; BUFFER WITH WEAK_PULLDOWN_ON AT 10% SUPPLY
|VARIATION WITH SC1=1 MEANING SLOW MODE OF OPERATION
BC40D_H_PU_ON_10P_!SC1_1P8  Cell operated at 1.8(nom)
|BC40D_H_PU_ON_10P_!SC1_1P8; BUFFER WITH WEAK_PULLUP_ON AT 10% SUPPLY
|VARIATION WITH SC1=0 MEANING FAST MODE OF OPERATION
BC40D_H_PUPDOFF_10P_!SC1_1P8  Cell operated at 1.8(nom)
|BC40D_H_PUPDOFF_10P_!SC1_1P8; BUFFER WITH WEAK PULUP/PULLDOWN OFF AT 10% SUPPLY
|VARIATION WITH SC1=0 MEANING FAST MODE OF OPERATION
BC40D_H_PU_ON_10P_SC1_1P8  Cell operated at 1.8(nom)
|BC40D_H_PU_ON_10P_SC1_1P8; BUFFER WITH WEAK_PULLUP_ON AT 10% SUPPLY
|VARIATION WITH SC1=1 MEANING SLOW MODE OF OPERATION
| 10% SUPPLY VARIATION MODES WITH 3.3V NOM SUPPLY
BC40D_H_PUPDOFF_10P_SC1_3P3  Cell operated at 3.3(nom)
|BC40D_H_PUPDOFF_10P_SC1_3P3; BUFFER WITH WEAK PULUP/PULLDOWN OFF AT 10% SUPPLY
|VARIATION WITH SC1=1 MEANING SLOW MODE OF OPERATION
BC40D_H_PD_ON_10P_!SC1_3P3  Cell operated at 3.3(nom)
|BC40D_H_PD_ON_10P_!SC1_3P3; BUFFER WITH WEAK_PULLDOWN_ON 10% SUPPLY
|VARIATION WITH SC1=0 MEANING FAST MODE OF OPERATION
BC40D_H_PD_ON_10P_SC1_3P3  Cell operated at 3.3(nom)
|BC40D_H_PD_ON_10P_SC1_3P3; BUFFER WITH WEAK_PULLDOWN_ON AT 10% SUPPLY
|VARIATION WITH SC1=1 MEANING SLOW MODE OF OPERATION
BC40D_H_PU_ON_10P_!SC1_3P3  Cell operated at 3.3(nom)
|BC40D_H_PU_ON_10P_!SC1_3P3; BUFFER WITH WEAK_PULLUP_ON AT 10% SUPPLY
|VARIATION WITH SC1=0 MEANING FAST MODE OF OPERATION
BC40D_H_PUPDOFF_10P_!SC1_3P3  Cell operated at 3.3(nom)
|BC40D_H_PUPDOFF_10P_!SC1_3P3; BUFFER WITH WEAK PULUP/PULLDOWN OFF AT 10% SUPPLY
|VARIATION WITH SC1=0 MEANING FAST MODE OF OPERATION
BC40D_H_PU_ON_10P_SC1_3P3  Cell operated at 3.3(nom)
|BC40D_H_PU_ON_10P_SC1_3P3; BUFFER WITH WEAK_PULLUP_ON AT 10% SUPPLY
|VARIATION WITH SC1=1 MEANING SLOW MODE OF OPERATION
|   BC1833DV40DCPBFBP18LL_RXLL_SSDLV
[Model Selector] bc1833dv40dcpbfbp18ll_rxll_ssdlv
|SC1 IS A SLEW RATE CONTROL PIN
|5% SUPPLY VARIATION MODES WITH 1.8V NOM SUPPLY
BC40D_V_PUPDOFF_5P_SC1_1P8  Cell operated at 1.8(nom)
|BC40D_V_PUPDOFF_5P_SC1_1P8; BUFFER WITH WEAK PULUP/PULLDOWN OFF AT 5% SUPPLY
|VARIATION WITH SC1=1 MEANING SLOW MODE OF OPERATION
BC40D_V_PD_ON_5P_!SC1_1P8  Cell operated at 1.8(nom)
|BC40D_V_PD_ON_5P_!SC1_1P8; BUFFER WITH WEAK_PULLDOWN_ON AT 5% SUPPLY
|VARIATION WITH SC1=0 MEANING FAST MODE OF OPERATION
BC40D_V_PD_ON_5P_SC1_1P8  Cell operated at 1.8(nom)
|BC40D_V_PD_ON_5P_SC1_1P8; BUFFER WITH WEAK_PULLDOWN_ON AT 5% SUPPLY
|VARIATION WITH SC1=1 MEANING SLOW MODE OF OPERATION
BC40D_V_PU_ON_5P_!SC1_1P8  Cell operated at 1.8(nom)
|BC40D_V_PU_ON_5P_!SC1_1P8; BUFFER WITH WEAK_PULLUP_ON AT 5% SUPPLY
|VARIATION WITH SC1=0 MEANING FAST MODE OF OPERATION
BC40D_V_PUPDOFF_5P_!SC1_1P8  Cell operated at 1.8(nom)
|BC40D_V_PUPDOFF_5P_!SC1_1P8; BUFFER WITH WEAK PULUP/PULLDOWN OFF AT 5% SUPPLY
|VARIATION WITH SC1=0 MEANING FAST MODE OF OPERATION
BC40D_V_PU_ON_5P_SC1_1P8  Cell operated at 1.8(nom)
|BC40D_V_PU_ON_5P_SC1_1P8; BUFFER WITH WEAK_PULLUP_ON AT 5% SUPPLY
|VARIATION WITH SC1=1 MEANING SLOW MODE OF OPERATION
|5% SUPPLY VARIATION MODES WITH 3.3V NOM SUPPLY
BC40D_V_PUPDOFF_5P_SC1_3P3  Cell operated at 3.3(nom)
|BC40D_V_PUPDOFF_5P_SC1_3P3; BUFFER WITH WEAK PULUP/PULLDOWN OFF AT 5% SUPPLY
|VARIATION WITH SC1=1 MEANING SLOW MODE OF OPERATION
BC40D_V_PD_ON_5P_!SC1_3P3  Cell operated at 3.3(nom)
|BC40D_V_PD_ON_5P_!SC1_3P3; BUFFER WITH WEAK_PULLDOWN_ON AT 5% SUPPLY
|VARIATION WITH SC1=0 MEANING FAST MODE OF OPERATION
BC40D_V_PD_ON_5P_SC1_3P3  Cell operated at 3.3(nom)
|BC40D_V_PD_ON_5P_SC1_3P3; BUFFER WITH WEAK_PULLDOWN_ON AT 5% SUPPLY
|VARIATION WITH SC1=1 MEANING SLOW MODE OF OPERATION
BC40D_V_PU_ON_5P_!SC1_3P3  Cell operated at 3.3(nom)
|BC40D_V_PU_ON_5P_!SC1_3P3; BUFFER WITH WEAK_PULLUP_ON AT 5% SUPPLY
|VARIATION WITH SC1=0 MEANING FAST MODE OF OPERATION
BC40D_V_PUPDOFF_5P_!SC1_3P3  Cell operated at 3.3(nom)
|BC40D_V_PUPDOFF_5P_!SC1_3P3; BUFFER WITH WEAK PULUP/PULLDOWN OFF AT 5% SUPPLY
|VARIATION WITH SC1=0 MEANING FAST MODE OF OPERATION
BC40D_V_PU_ON_5P_SC1_3P3  Cell operated at 3.3(nom)
|BC40D_V_PU_ON_5P_SC1_3P3; BUFFER WITH WEAK_PULLUP_ON AT 5% SUPPLY
|VARIATION WITH SC1=1 MEANING SLOW MODE OF OPERATION
| 10% SUPPLY VARIATION MODES WITH 1.8V NOM SUPPLY
BC40D_V_PUPDOFF_10P_SC1_1P8  Cell operated at 1.8(nom)
|BC40D_V_PUPDOFF_10P_SC1_1P8; BUFFER WITH WEAK PULUP/PULLDOWN OFF AT 10% SUPPLY
|VARIATION WITH SC1=1 MEANING SLOW MODE OF OPERATION
BC40D_V_PD_ON_10P_!SC1_1P8  Cell operated at 1.8(nom)
|BC40D_V_PD_ON_10P_!SC1_1P8; BUFFER WITH WEAK_PULLDOWN_ON AT 10% SUPPLY
|VARIATION WITH SC1=0 MEANING FAST MODE OF OPERATION
BC40D_V_PD_ON_10P_SC1_1P8  Cell operated at 1.8(nom)
|BC40D_V_PD_ON_10P_SC1_1P8; BUFFER WITH WEAK_PULLDOWN_ON AT 10% SUPPLY
|VARIATION WITH SC1=1 MEANING SLOW MODE OF OPERATION
BC40D_V_PU_ON_10P_!SC1_1P8  Cell operated at 1.8(nom)
|BC40D_V_PU_ON_10P_!SC1_1P8; BUFFER WITH WEAK_PULLUP_ON AT 10% SUPPLY
|VARIATION WITH SC1=0 MEANING FAST MODE OF OPERATION
BC40D_V_PUPDOFF_10P_!SC1_1P8  Cell operated at 1.8(nom)
|BC40D_V_PUPDOFF_10P_!SC1_1P8; BUFFER WITH WEAK PULUP/PULLDOWN OFF AT 10% SUPPLY
|VARIATION WITH SC1=0 MEANING FAST MODE OF OPERATION
BC40D_V_PU_ON_10P_SC1_1P8  Cell operated at 1.8(nom)
|BC40D_V_PU_ON_10P_SC1_1P8; BUFFER WITH WEAK_PULLUP_ON AT 10% SUPPLY
|VARIATION WITH SC1=1 MEANING SLOW MODE OF OPERATION
| 10% SUPPLY VARIATION MODES WITH 3.3V NOM SUPPLY
BC40D_V_PUPDOFF_10P_SC1_3P3  Cell operated at 3.3(nom)
|BC40D_V_PUPDOFF_10P_SC1_3P3; BUFFER WITH WEAK PULUP/PULLDOWN OFF AT 10% SUPPLY
|VARIATION WITH SC1=1 MEANING SLOW MODE OF OPERATION
BC40D_V_PD_ON_10P_!SC1_3P3  Cell operated at 3.3(nom)
|BC40D_V_PD_ON_10P_!SC1_3P3; BUFFER WITH WEAK_PULLDOWN_ON 10% SUPPLY
|VARIATION WITH SC1=0 MEANING FAST MODE OF OPERATION
BC40D_V_PD_ON_10P_SC1_3P3  Cell operated at 3.3(nom)
|BC40D_V_PD_ON_10P_SC1_3P3; BUFFER WITH WEAK_PULLDOWN_ON AT 10% SUPPLY
|VARIATION WITH SC1=1 MEANING SLOW MODE OF OPERATION
BC40D_V_PU_ON_10P_!SC1_3P3  Cell operated at 3.3(nom)
|BC40D_V_PU_ON_10P_!SC1_3P3; BUFFER WITH WEAK_PULLUP_ON AT 10% SUPPLY
|VARIATION WITH SC1=0 MEANING FAST MODE OF OPERATION
BC40D_V_PUPDOFF_10P_!SC1_3P3  Cell operated at 3.3(nom)
|BC40D_V_PUPDOFF_10P_!SC1_3P3; BUFFER WITH WEAK PULUP/PULLDOWN OFF AT 10% SUPPLY
|VARIATION WITH SC1=0 MEANING FAST MODE OF OPERATION
BC40D_V_PU_ON_10P_SC1_3P3  Cell operated at 3.3(nom)
|BC40D_V_PU_ON_10P_SC1_3P3; BUFFER WITH WEAK_PULLUP_ON AT 10% SUPPLY
|VARIATION WITH SC1=1 MEANING SLOW MODE OF OPERATION
|   BC1833DV40DCPBFBP18LL_RXLL_SSDLH_135U
[Model Selector] bc1833dv40dcpbfbp18ll_rxll_ssdlh_135u
|SC1 IS A SLEW RATE CONTROL PIN
|5% SUPPLY VARIATION MODES WITH 1.8V NOM SUPPLY
BC40D_H_PUPDOFF_5P_SC1_1P8  Cell operated at 1.8(nom)
|BC40D_H_PUPDOFF_5P_SC1_1P8; BUFFER WITH WEAK PULUP/PULLDOWN OFF AT 5% SUPPLY
|VARIATION WITH SC1=1 MEANING SLOW MODE OF OPERATION
BC40D_H_PD_ON_5P_!SC1_1P8  Cell operated at 1.8(nom)
|BC40D_H_PD_ON_5P_!SC1_1P8; BUFFER WITH WEAK_PULLDOWN_ON AT 5% SUPPLY
|VARIATION WITH SC1=0 MEANING FAST MODE OF OPERATION
BC40D_H_PD_ON_5P_SC1_1P8  Cell operated at 1.8(nom)
|BC40D_H_PD_ON_5P_SC1_1P8; BUFFER WITH WEAK_PULLDOWN_ON AT 5% SUPPLY
|VARIATION WITH SC1=1 MEANING SLOW MODE OF OPERATION
BC40D_H_PU_ON_5P_!SC1_1P8  Cell operated at 1.8(nom)
|BC40D_H_PU_ON_5P_!SC1_1P8; BUFFER WITH WEAK_PULLUP_ON AT 5% SUPPLY
|VARIATION WITH SC1=0 MEANING FAST MODE OF OPERATION
BC40D_H_PUPDOFF_5P_!SC1_1P8  Cell operated at 1.8(nom)
|BC40D_H_PUPDOFF_5P_!SC1_1P8; BUFFER WITH WEAK PULUP/PULLDOWN OFF AT 5% SUPPLY
|VARIATION WITH SC1=0 MEANING FAST MODE OF OPERATION
BC40D_H_PU_ON_5P_SC1_1P8  Cell operated at 1.8(nom)
|BC40D_H_PU_ON_5P_SC1_1P8; BUFFER WITH WEAK_PULLUP_ON AT 5% SUPPLY
|VARIATION WITH SC1=1 MEANING SLOW MODE OF OPERATION
|5% SUPPLY VARIATION MODES WITH 3.3V NOM SUPPLY
BC40D_H_PUPDOFF_5P_SC1_3P3  Cell operated at 3.3(nom)
|BC40D_H_PUPDOFF_5P_SC1_3P3; BUFFER WITH WEAK PULUP/PULLDOWN OFF AT 5% SUPPLY
|VARIATION WITH SC1=1 MEANING SLOW MODE OF OPERATION
BC40D_H_PD_ON_5P_!SC1_3P3  Cell operated at 3.3(nom)
|BC40D_H_PD_ON_5P_!SC1_3P3; BUFFER WITH WEAK_PULLDOWN_ON AT 5% SUPPLY
|VARIATION WITH SC1=0 MEANING FAST MODE OF OPERATION
BC40D_H_PD_ON_5P_SC1_3P3  Cell operated at 3.3(nom)
|BC40D_H_PD_ON_5P_SC1_3P3; BUFFER WITH WEAK_PULLDOWN_ON AT 5% SUPPLY
|VARIATION WITH SC1=1 MEANING SLOW MODE OF OPERATION
BC40D_H_PU_ON_5P_!SC1_3P3  Cell operated at 3.3(nom)
|BC40D_H_PU_ON_5P_!SC1_3P3; BUFFER WITH WEAK_PULLUP_ON AT 5% SUPPLY
|VARIATION WITH SC1=0 MEANING FAST MODE OF OPERATION
BC40D_H_PUPDOFF_5P_!SC1_3P3  Cell operated at 3.3(nom)
|BC40D_H_PUPDOFF_5P_!SC1_3P3; BUFFER WITH WEAK PULUP/PULLDOWN OFF AT 5% SUPPLY
|VARIATION WITH SC1=0 MEANING FAST MODE OF OPERATION
BC40D_H_PU_ON_5P_SC1_3P3  Cell operated at 3.3(nom)
|BC40D_H_PU_ON_5P_SC1_3P3; BUFFER WITH WEAK_PULLUP_ON AT 5% SUPPLY
|VARIATION WITH SC1=1 MEANING SLOW MODE OF OPERATION
| 10% SUPPLY VARIATION MODES WITH 1.8V NOM SUPPLY
BC40D_H_PUPDOFF_10P_SC1_1P8  Cell operated at 1.8(nom)
|BC40D_H_PUPDOFF_10P_SC1_1P8; BUFFER WITH WEAK PULUP/PULLDOWN OFF AT 10% SUPPLY
|VARIATION WITH SC1=1 MEANING SLOW MODE OF OPERATION
BC40D_H_PD_ON_10P_!SC1_1P8  Cell operated at 1.8(nom)
|BC40D_H_PD_ON_10P_!SC1_1P8; BUFFER WITH WEAK_PULLDOWN_ON AT 10% SUPPLY
|VARIATION WITH SC1=0 MEANING FAST MODE OF OPERATION
BC40D_H_PD_ON_10P_SC1_1P8  Cell operated at 1.8(nom)
|BC40D_H_PD_ON_10P_SC1_1P8; BUFFER WITH WEAK_PULLDOWN_ON AT 10% SUPPLY
|VARIATION WITH SC1=1 MEANING SLOW MODE OF OPERATION
BC40D_H_PU_ON_10P_!SC1_1P8  Cell operated at 1.8(nom)
|BC40D_H_PU_ON_10P_!SC1_1P8; BUFFER WITH WEAK_PULLUP_ON AT 10% SUPPLY
|VARIATION WITH SC1=0 MEANING FAST MODE OF OPERATION
BC40D_H_PUPDOFF_10P_!SC1_1P8  Cell operated at 1.8(nom)
|BC40D_H_PUPDOFF_10P_!SC1_1P8; BUFFER WITH WEAK PULUP/PULLDOWN OFF AT 10% SUPPLY
|VARIATION WITH SC1=0 MEANING FAST MODE OF OPERATION
BC40D_H_PU_ON_10P_SC1_1P8  Cell operated at 1.8(nom)
|BC40D_H_PU_ON_10P_SC1_1P8; BUFFER WITH WEAK_PULLUP_ON AT 10% SUPPLY
|VARIATION WITH SC1=1 MEANING SLOW MODE OF OPERATION
| 10% SUPPLY VARIATION MODES WITH 3.3V NOM SUPPLY
BC40D_H_PUPDOFF_10P_SC1_3P3  Cell operated at 3.3(nom)
|BC40D_H_PUPDOFF_10P_SC1_3P3; BUFFER WITH WEAK PULUP/PULLDOWN OFF AT 10% SUPPLY
|VARIATION WITH SC1=1 MEANING SLOW MODE OF OPERATION
BC40D_H_PD_ON_10P_!SC1_3P3  Cell operated at 3.3(nom)
|BC40D_H_PD_ON_10P_!SC1_3P3; BUFFER WITH WEAK_PULLDOWN_ON 10% SUPPLY
|VARIATION WITH SC1=0 MEANING FAST MODE OF OPERATION
BC40D_H_PD_ON_10P_SC1_3P3  Cell operated at 3.3(nom)
|BC40D_H_PD_ON_10P_SC1_3P3; BUFFER WITH WEAK_PULLDOWN_ON AT 10% SUPPLY
|VARIATION WITH SC1=1 MEANING SLOW MODE OF OPERATION
BC40D_H_PU_ON_10P_!SC1_3P3  Cell operated at 3.3(nom)
|BC40D_H_PU_ON_10P_!SC1_3P3; BUFFER WITH WEAK_PULLUP_ON AT 10% SUPPLY
|VARIATION WITH SC1=0 MEANING FAST MODE OF OPERATION
BC40D_H_PUPDOFF_10P_!SC1_3P3  Cell operated at 3.3(nom)
|BC40D_H_PUPDOFF_10P_!SC1_3P3; BUFFER WITH WEAK PULUP/PULLDOWN OFF AT 10% SUPPLY
|VARIATION WITH SC1=0 MEANING FAST MODE OF OPERATION
BC40D_H_PU_ON_10P_SC1_3P3  Cell operated at 3.3(nom)
|BC40D_H_PU_ON_10P_SC1_3P3; BUFFER WITH WEAK_PULLUP_ON AT 10% SUPPLY
|VARIATION WITH SC1=1 MEANING SLOW MODE OF OPERATION
|   BC1833DV40DCPBFBP18LL_RXLL_SSDLV_135U
[Model Selector] bc1833dv40dcpbfbp18ll_rxll_ssdlv_135u
|SC1 IS A SLEW RATE CONTROL PIN
|5% SUPPLY VARIATION MODES WITH 1.8V NOM SUPPLY
BC40D_V_PUPDOFF_5P_SC1_1P8  Cell operated at 1.8(nom)
|BC40D_V_PUPDOFF_5P_SC1_1P8; BUFFER WITH WEAK PULUP/PULLDOWN OFF AT 5% SUPPLY
|VARIATION WITH SC1=1 MEANING SLOW MODE OF OPERATION
BC40D_V_PD_ON_5P_!SC1_1P8  Cell operated at 1.8(nom)
|BC40D_V_PD_ON_5P_!SC1_1P8; BUFFER WITH WEAK_PULLDOWN_ON AT 5% SUPPLY
|VARIATION WITH SC1=0 MEANING FAST MODE OF OPERATION
BC40D_V_PD_ON_5P_SC1_1P8  Cell operated at 1.8(nom)
|BC40D_V_PD_ON_5P_SC1_1P8; BUFFER WITH WEAK_PULLDOWN_ON AT 5% SUPPLY
|VARIATION WITH SC1=1 MEANING SLOW MODE OF OPERATION
BC40D_V_PU_ON_5P_!SC1_1P8  Cell operated at 1.8(nom)
|BC40D_V_PU_ON_5P_!SC1_1P8; BUFFER WITH WEAK_PULLUP_ON AT 5% SUPPLY
|VARIATION WITH SC1=0 MEANING FAST MODE OF OPERATION
BC40D_V_PUPDOFF_5P_!SC1_1P8  Cell operated at 1.8(nom)
|BC40D_V_PUPDOFF_5P_!SC1_1P8; BUFFER WITH WEAK PULUP/PULLDOWN OFF AT 5% SUPPLY
|VARIATION WITH SC1=0 MEANING FAST MODE OF OPERATION
BC40D_V_PU_ON_5P_SC1_1P8  Cell operated at 1.8(nom)
|BC40D_V_PU_ON_5P_SC1_1P8; BUFFER WITH WEAK_PULLUP_ON AT 5% SUPPLY
|VARIATION WITH SC1=1 MEANING SLOW MODE OF OPERATION
|5% SUPPLY VARIATION MODES WITH 3.3V NOM SUPPLY
BC40D_V_PUPDOFF_5P_SC1_3P3  Cell operated at 3.3(nom)
|BC40D_V_PUPDOFF_5P_SC1_3P3; BUFFER WITH WEAK PULUP/PULLDOWN OFF AT 5% SUPPLY
|VARIATION WITH SC1=1 MEANING SLOW MODE OF OPERATION
BC40D_V_PD_ON_5P_!SC1_3P3  Cell operated at 3.3(nom)
|BC40D_V_PD_ON_5P_!SC1_3P3; BUFFER WITH WEAK_PULLDOWN_ON AT 5% SUPPLY
|VARIATION WITH SC1=0 MEANING FAST MODE OF OPERATION
BC40D_V_PD_ON_5P_SC1_3P3  Cell operated at 3.3(nom)
|BC40D_V_PD_ON_5P_SC1_3P3; BUFFER WITH WEAK_PULLDOWN_ON AT 5% SUPPLY
|VARIATION WITH SC1=1 MEANING SLOW MODE OF OPERATION
BC40D_V_PU_ON_5P_!SC1_3P3  Cell operated at 3.3(nom)
|BC40D_V_PU_ON_5P_!SC1_3P3; BUFFER WITH WEAK_PULLUP_ON AT 5% SUPPLY
|VARIATION WITH SC1=0 MEANING FAST MODE OF OPERATION
BC40D_V_PUPDOFF_5P_!SC1_3P3  Cell operated at 3.3(nom)
|BC40D_V_PUPDOFF_5P_!SC1_3P3; BUFFER WITH WEAK PULUP/PULLDOWN OFF AT 5% SUPPLY
|VARIATION WITH SC1=0 MEANING FAST MODE OF OPERATION
BC40D_V_PU_ON_5P_SC1_3P3  Cell operated at 3.3(nom)
|BC40D_V_PU_ON_5P_SC1_3P3; BUFFER WITH WEAK_PULLUP_ON AT 5% SUPPLY
|VARIATION WITH SC1=1 MEANING SLOW MODE OF OPERATION
| 10% SUPPLY VARIATION MODES WITH 1.8V NOM SUPPLY
BC40D_V_PUPDOFF_10P_SC1_1P8  Cell operated at 1.8(nom)
|BC40D_V_PUPDOFF_10P_SC1_1P8; BUFFER WITH WEAK PULUP/PULLDOWN OFF AT 10% SUPPLY
|VARIATION WITH SC1=1 MEANING SLOW MODE OF OPERATION
BC40D_V_PD_ON_10P_!SC1_1P8  Cell operated at 1.8(nom)
|BC40D_V_PD_ON_10P_!SC1_1P8; BUFFER WITH WEAK_PULLDOWN_ON AT 10% SUPPLY
|VARIATION WITH SC1=0 MEANING FAST MODE OF OPERATION
BC40D_V_PD_ON_10P_SC1_1P8  Cell operated at 1.8(nom)
|BC40D_V_PD_ON_10P_SC1_1P8; BUFFER WITH WEAK_PULLDOWN_ON AT 10% SUPPLY
|VARIATION WITH SC1=1 MEANING SLOW MODE OF OPERATION
BC40D_V_PU_ON_10P_!SC1_1P8  Cell operated at 1.8(nom)
|BC40D_V_PU_ON_10P_!SC1_1P8; BUFFER WITH WEAK_PULLUP_ON AT 10% SUPPLY
|VARIATION WITH SC1=0 MEANING FAST MODE OF OPERATION
BC40D_V_PUPDOFF_10P_!SC1_1P8  Cell operated at 1.8(nom)
|BC40D_V_PUPDOFF_10P_!SC1_1P8; BUFFER WITH WEAK PULUP/PULLDOWN OFF AT 10% SUPPLY
|VARIATION WITH SC1=0 MEANING FAST MODE OF OPERATION
BC40D_V_PU_ON_10P_SC1_1P8  Cell operated at 1.8(nom)
|BC40D_V_PU_ON_10P_SC1_1P8; BUFFER WITH WEAK_PULLUP_ON AT 10% SUPPLY
|VARIATION WITH SC1=1 MEANING SLOW MODE OF OPERATION
| 10% SUPPLY VARIATION MODES WITH 3.3V NOM SUPPLY
BC40D_V_PUPDOFF_10P_SC1_3P3  Cell operated at 3.3(nom)
|BC40D_V_PUPDOFF_10P_SC1_3P3; BUFFER WITH WEAK PULUP/PULLDOWN OFF AT 10% SUPPLY
|VARIATION WITH SC1=1 MEANING SLOW MODE OF OPERATION
BC40D_V_PD_ON_10P_!SC1_3P3  Cell operated at 3.3(nom)
|BC40D_V_PD_ON_10P_!SC1_3P3; BUFFER WITH WEAK_PULLDOWN_ON 10% SUPPLY
|VARIATION WITH SC1=0 MEANING FAST MODE OF OPERATION
BC40D_V_PD_ON_10P_SC1_3P3  Cell operated at 3.3(nom)
|BC40D_V_PD_ON_10P_SC1_3P3; BUFFER WITH WEAK_PULLDOWN_ON AT 10% SUPPLY
|VARIATION WITH SC1=1 MEANING SLOW MODE OF OPERATION
BC40D_V_PU_ON_10P_!SC1_3P3  Cell operated at 3.3(nom)
|BC40D_V_PU_ON_10P_!SC1_3P3; BUFFER WITH WEAK_PULLUP_ON AT 10% SUPPLY
|VARIATION WITH SC1=0 MEANING FAST MODE OF OPERATION
BC40D_V_PUPDOFF_10P_!SC1_3P3  Cell operated at 3.3(nom)
|BC40D_V_PUPDOFF_10P_!SC1_3P3; BUFFER WITH WEAK PULUP/PULLDOWN OFF AT 10% SUPPLY
|VARIATION WITH SC1=0 MEANING FAST MODE OF OPERATION
BC40D_V_PU_ON_10P_SC1_3P3  Cell operated at 3.3(nom)
|BC40D_V_PU_ON_10P_SC1_3P3; BUFFER WITH WEAK_PULLUP_ON AT 10% SUPPLY
|VARIATION WITH SC1=1 MEANING SLOW MODE OF OPERATION
|   BC1833DV40DCPBFBP18LL_SSDLH_135U
[Model Selector] bc1833dv40dcpbfbp18ll_ssdlh_135u
|SC1 IS A SLEW RATE CONTROL PIN
|5% SUPPLY VARIATION MODES WITH 1.8V NOM SUPPLY
BC40D_H_PUPDOFF_5P_SC1_1P8  Cell operated at 1.8(nom)
|BC40D_H_PUPDOFF_5P_SC1_1P8; BUFFER WITH WEAK PULUP/PULLDOWN OFF AT 5% SUPPLY
|VARIATION WITH SC1=1 MEANING SLOW MODE OF OPERATION
BC40D_H_PD_ON_5P_!SC1_1P8  Cell operated at 1.8(nom)
|BC40D_H_PD_ON_5P_!SC1_1P8; BUFFER WITH WEAK_PULLDOWN_ON AT 5% SUPPLY
|VARIATION WITH SC1=0 MEANING FAST MODE OF OPERATION
BC40D_H_PD_ON_5P_SC1_1P8  Cell operated at 1.8(nom)
|BC40D_H_PD_ON_5P_SC1_1P8; BUFFER WITH WEAK_PULLDOWN_ON AT 5% SUPPLY
|VARIATION WITH SC1=1 MEANING SLOW MODE OF OPERATION
BC40D_H_PU_ON_5P_!SC1_1P8  Cell operated at 1.8(nom)
|BC40D_H_PU_ON_5P_!SC1_1P8; BUFFER WITH WEAK_PULLUP_ON AT 5% SUPPLY
|VARIATION WITH SC1=0 MEANING FAST MODE OF OPERATION
BC40D_H_PUPDOFF_5P_!SC1_1P8  Cell operated at 1.8(nom)
|BC40D_H_PUPDOFF_5P_!SC1_1P8; BUFFER WITH WEAK PULUP/PULLDOWN OFF AT 5% SUPPLY
|VARIATION WITH SC1=0 MEANING FAST MODE OF OPERATION
BC40D_H_PU_ON_5P_SC1_1P8  Cell operated at 1.8(nom)
|BC40D_H_PU_ON_5P_SC1_1P8; BUFFER WITH WEAK_PULLUP_ON AT 5% SUPPLY
|VARIATION WITH SC1=1 MEANING SLOW MODE OF OPERATION
|5% SUPPLY VARIATION MODES WITH 3.3V NOM SUPPLY
BC40D_H_PUPDOFF_5P_SC1_3P3  Cell operated at 3.3(nom)
|BC40D_H_PUPDOFF_5P_SC1_3P3; BUFFER WITH WEAK PULUP/PULLDOWN OFF AT 5% SUPPLY
|VARIATION WITH SC1=1 MEANING SLOW MODE OF OPERATION
BC40D_H_PD_ON_5P_!SC1_3P3  Cell operated at 3.3(nom)
|BC40D_H_PD_ON_5P_!SC1_3P3; BUFFER WITH WEAK_PULLDOWN_ON AT 5% SUPPLY
|VARIATION WITH SC1=0 MEANING FAST MODE OF OPERATION
BC40D_H_PD_ON_5P_SC1_3P3  Cell operated at 3.3(nom)
|BC40D_H_PD_ON_5P_SC1_3P3; BUFFER WITH WEAK_PULLDOWN_ON AT 5% SUPPLY
|VARIATION WITH SC1=1 MEANING SLOW MODE OF OPERATION
BC40D_H_PU_ON_5P_!SC1_3P3  Cell operated at 3.3(nom)
|BC40D_H_PU_ON_5P_!SC1_3P3; BUFFER WITH WEAK_PULLUP_ON AT 5% SUPPLY
|VARIATION WITH SC1=0 MEANING FAST MODE OF OPERATION
BC40D_H_PUPDOFF_5P_!SC1_3P3  Cell operated at 3.3(nom)
|BC40D_H_PUPDOFF_5P_!SC1_3P3; BUFFER WITH WEAK PULUP/PULLDOWN OFF AT 5% SUPPLY
|VARIATION WITH SC1=0 MEANING FAST MODE OF OPERATION
BC40D_H_PU_ON_5P_SC1_3P3  Cell operated at 3.3(nom)
|BC40D_H_PU_ON_5P_SC1_3P3; BUFFER WITH WEAK_PULLUP_ON AT 5% SUPPLY
|VARIATION WITH SC1=1 MEANING SLOW MODE OF OPERATION
| 10% SUPPLY VARIATION MODES WITH 1.8V NOM SUPPLY
BC40D_H_PUPDOFF_10P_SC1_1P8  Cell operated at 1.8(nom)
|BC40D_H_PUPDOFF_10P_SC1_1P8; BUFFER WITH WEAK PULUP/PULLDOWN OFF AT 10% SUPPLY
|VARIATION WITH SC1=1 MEANING SLOW MODE OF OPERATION
BC40D_H_PD_ON_10P_!SC1_1P8  Cell operated at 1.8(nom)
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| Models and submodels in the file (68): BC40D_H_PUPDOFF_5P_SC1_1P8 (I/O), BC40D_H_PD_ON_5P_!SC1_1P8 (I/O), BC40D_H_PD_ON_5P_SC1_1P8 (I/O), BC40D_H_PU_ON_5P_!SC1_1P8 (I/O), BC40D_H_PUPDOFF_5P_!SC1_1P8 (I/O), BC40D_H_PU_ON_5P_SC1_1P8 (I/O), BC40D_H_PUPDOFF_5P_SC1_3P3 (I/O), BC40D_H_PD_ON_5P_!SC1_3P3 (I/O), BC40D_H_PD_ON_5P_SC1_3P3 (I/O), BC40D_H_PU_ON_5P_!SC1_3P3 (I/O), BC40D_H_PUPDOFF_5P_!SC1_3P3 (I/O), BC40D_H_PU_ON_5P_SC1_3P3 (I/O), BC40D_H_PUPDOFF_10P_SC1_1P8 (I/O), BC40D_H_PD_ON_10P_!SC1_1P8 (I/O), BC40D_H_PD_ON_10P_SC1_1P8 (I/O), BC40D_H_PU_ON_10P_!SC1_1P8 (I/O), BC40D_H_PUPDOFF_10P_!SC1_1P8 (I/O), BC40D_H_PU_ON_10P_SC1_1P8 (I/O), BC40D_H_PUPDOFF_10P_SC1_3P3 (I/O), BC40D_H_PD_ON_10P_!SC1_3P3 (I/O), BC40D_H_PD_ON_10P_SC1_3P3 (I/O), BC40D_H_PU_ON_10P_!SC1_3P3 (I/O), BC40D_H_PUPDOFF_10P_!SC1_3P3 (I/O), BC40D_H_PU_ON_10P_SC1_3P3 (I/O), BC40D_V_PUPDOFF_5P_SC1_1P8 (I/O), BC40D_V_PD_ON_5P_!SC1_1P8 (I/O), BC40D_V_PD_ON_5P_SC1_1P8 (I/O), BC40D_V_PU_ON_5P_!SC1_1P8 (I/O), BC40D_V_PUPDOFF_5P_!SC1_1P8 (I/O), BC40D_V_PU_ON_5P_SC1_1P8 (I/O), BC40D_V_PUPDOFF_5P_SC1_3P3 (I/O), BC40D_V_PD_ON_5P_!SC1_3P3 (I/O), BC40D_V_PD_ON_5P_SC1_3P3 (I/O), BC40D_V_PU_ON_5P_!SC1_3P3 (I/O), BC40D_V_PUPDOFF_5P_!SC1_3P3 (I/O), BC40D_V_PU_ON_5P_SC1_3P3 (I/O), BC40D_V_PUPDOFF_10P_SC1_1P8 (I/O), BC40D_V_PD_ON_10P_!SC1_1P8 (I/O), BC40D_V_PD_ON_10P_SC1_1P8 (I/O), BC40D_V_PU_ON_10P_!SC1_1P8 (I/O), BC40D_V_PUPDOFF_10P_!SC1_1P8 (I/O), BC40D_V_PU_ON_10P_SC1_1P8 (I/O), BC40D_V_PUPDOFF_10P_SC1_3P3 (I/O), BC40D_V_PD_ON_10P_!SC1_3P3 (I/O), BC40D_V_PD_ON_10P_SC1_3P3 (I/O), BC40D_V_PU_ON_10P_!SC1_3P3 (I/O), BC40D_V_PUPDOFF_10P_!SC1_3P3 (I/O), BC40D_V_PU_ON_10P_SC1_3P3 (I/O), BI2C1833_NORAML_5P_1P8 (I/O_open_drain), BI2C1833_NORAML_5P_3P3 (I/O_open_drain), BI2C1833_NORAML_10P_1P8 (I/O_open_drain), BI2C1833_NORAML_10P_3P3 (I/O_open_drain), IHHV_NORAML_5P_1P8 (Input), IHHV_NORAML_5P_3P3 (Input), IHHV_NORAML_10P_1P8 (Input), IHHV_NORAML_10P_3P3 (Input), IQ_SSDHH_PD_ON_5P_1P8 (Input), IQ_SSDHH_PU_ON_5P_1P8 (Input), IQ_SSDHH_PUPDOFF_5P_1P8 (Input), IQ_SSDHH_PD_ON_5P_3P3 (Input), IQ_SSDHH_PU_ON_5P_3P3 (Input), IQ_SSDHH_PUPDOFF_5P_3P3 (Input), IQ_SSDHH_PD_ON_10P_1P8 (Input), IQ_SSDHH_PU_ON_10P_1P8 (Input), IQ_SSDHH_PUPDOFF_10P_1P8 (Input), IQ_SSDHH_PD_ON_10P_3P3 (Input), IQ_SSDHH_PU_ON_10P_3P3 (Input), IQ_SSDHH_PUPDOFF_10P_3P3 (Input)
